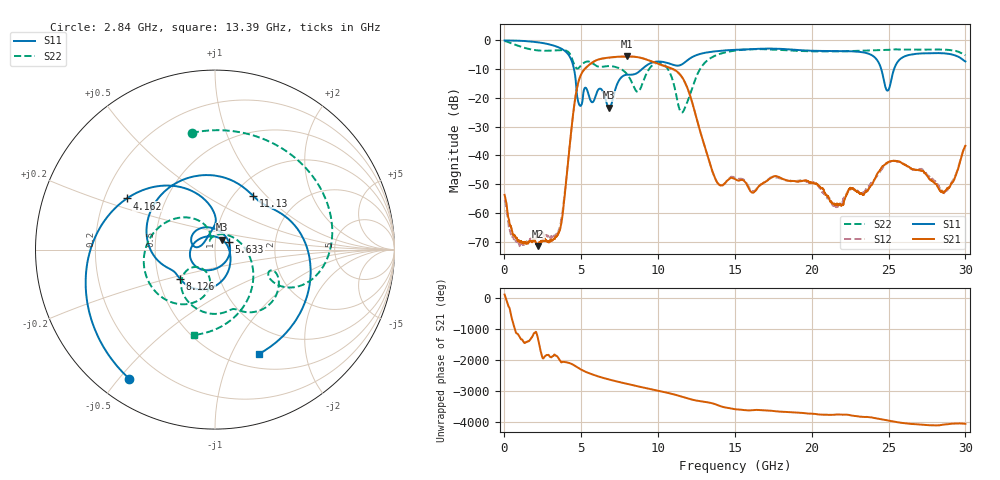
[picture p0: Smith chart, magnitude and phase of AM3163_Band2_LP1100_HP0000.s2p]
!Agilent Technologies,E8364B,MY43040894,A.07.50.67
!Agilent E8364B: A.07.50.67
!Date: Thursday, August 20, 2020 12:03:02
!Correction: S11(Full 2 Port(1,2))
!S21(Full 2 Port(1,2))
!S12(Full 2 Port(1,2))
!S22(Full 2 Port(1,2))
!S2P File: Measurements: S11, S21, S12, S22:
# Hz S  dB  R 50
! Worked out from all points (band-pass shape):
!   3201 points, 10 MHz to 30 GHz, reference 50 ohm
!   highest |S21| = -5.58 dB at 7.976 GHz (marker M1); lowest = -71.5 dB at 2.184 GHz (marker M2)
!   |S21| within 3 dB of the highest: 5.494 GHz to 10.26 GHz (4.766 GHz wide, 60.5 % of centre)
!   lowest |S11| = -23.4 dB at 6.814 GHz (marker M3), VSWR 1.15, Z = 53.8 + j5.95 ohm
!   |S11| at or under -10 dB: 4.528 GHz to 8.949 GHz (4.421 GHz wide, 65.6 % of centre); 24.52 GHz to 25.36 GHz (830.9 MHz wide, 3.33 % of centre)
!   |S22| runs from -25.1 to -0.2 dB; largest |S21 - S12| = 0.0054
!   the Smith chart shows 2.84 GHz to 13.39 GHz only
!   S11 on the Smith chart (normalised r, x): 2.84 GHz: 0.09, -0.53; 4.162 GHz: 0.29, +0.25; 5.633 GHz: 1.16, +0.09; 8.126 GHz: 0.64, -0.22; 11.13 GHz: 1.21, +0.84; 13.39 GHz: 0.66, -1.28
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1e7  -0.01 -2.9  -53.70 96.7  -55.45 -167.0  -0.21 -8.5
8.34725e8  -0.09 -34.5  -69.53 -76.2  -69.91 33.0  -1.75 -93.1
2.184275e9  -0.66 -92.6  -71.50 118.9  -68.26 -31.3  -3.47 150.2
2.840306e9  -1.27 -123.5  -70.01 -34.2  -67.90 -107.3  -3.57 101.3
3.627544e9  -2.65 -167.8  -65.58 138.1  -64.22 31.8  -3.35 42.8
4.161741e9  -4.92 149.9  -40.93 72.3  -40.97 71.7  -4.03 -4.1
5.014581e9  -22.36 157.9  -11.55 -152.4  -11.55 -152.7  -8.44 -22.7
5.633125e9  -21.16 27.5  -7.99 74.8  -8.03 74.5  -7.63 -56.1
6.813981e9  -23.36 54.1  -5.95 -104.2  -5.99 -104.3  -8.91 -90.8
7.976094e9  -11.92 -132.0  -5.58 117.5  -5.58 117.7  -11.72 -136.5
8.126044e9  -11.90 -140.0  -5.59 100.6  -5.58 100.8  -12.89 -141.3
8.978884e9  -9.86 -168.5  -6.19 5.2  -6.17 5.0  -15.02 -99.0
1.000979e10  -7.34 125.7  -8.14 -104.3  -8.24 -104.7  -7.73 -154.0
1.112504e10  -8.69 55.0  -10.41 127.2  -10.52 127.3  -17.58 109.7
1.339304e10  -4.00 -67.4  -43.09 -129.8  -43.18 -128.1  -6.22 -103.6
1.5005e10  -3.24 -138.1  -48.20 24.6  -47.74 25.8  -3.54 178.2
1.780719e10  -2.89 97.0  -47.44 -46.4  -47.71 -46.4  -3.26 59.8
2.000958e10  -3.59 -14.4  -49.44 -116.6  -49.59 -121.9  -3.79 -29.1
2.347718e10  -4.27 -148.9  -52.88 136.9  -52.17 139.5  -3.53 -134.3
2.500479e10  -17.12 -151.8  -42.27 17.3  -42.28 19.4  -3.31 -172.7
2.864108e10  -4.50 99.3  -52.67 -105.6  -53.07 -103.4  -3.21 91.1
3e10  -7.31 47.4  -36.66 -81.9  -36.53 -80.8  -5.14 50.7
